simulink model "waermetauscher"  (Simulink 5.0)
settings: Solver=ode45  StartTime=0.0  StopTime=Te  RelTol=1e-3
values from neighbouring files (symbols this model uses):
  A = [0 -1/L; 1/C 0]    [Aufgwok.m]    (also in Behalt.m = [-0.5 0; Bspkran.m = zeros(n, n); Bspmotor.m = [-RA/LA  -km/LA; Bsppend.m = [0  0        1        0)
  c1 = [1 0 0]    [Bsppend.m]    (also in BspSchwinger.m = 0.75; carbrklin.m = 1.2801)
  c2 = 0.4    [BspSchwinger.m]    (also in carbrklin.m = 23.99)
  dt = 0.03    [BodeInterpr.m]    (also in carbrklin.m = 0.01; PerfregSchwinger.m = 0.1; PerfregSchwingkreis.m = 0.0002)
  k = k+1    (= 1)    [Airbag.m]    (also in Bodedia.m = 2; Deltah.m; Fklmotr.m; Laplace.m = 0)
  m1 = 1    [Bsppend.m]    (also in BspSchwinger.m)
  m2 = 1    [BspSchwinger.m]
  w1 = 0.1    [BodeInterpr.m]    (also in FKLLeerlauf.m = 16.7833109017)
  w2 = 1    [BodeInterpr.m]
undefined symbols (not defined in the file or in its folder): deltad, deltaw, T10, T1quer, T20, T2quer

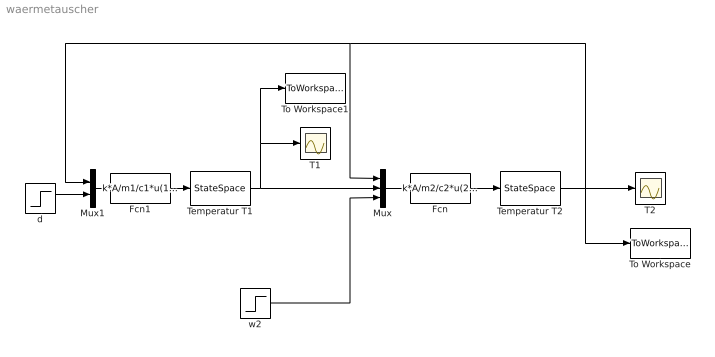
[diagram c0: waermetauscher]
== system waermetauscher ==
  Fcn : Fcn  Expr=k*A/m2/c2*u(2)+T20/m2*u(3)-u(1)*u(3)/m2
  Fcn1 : Fcn  Expr=k*A/m1/c1*u(1)+w1/m1*T10+w1/m1*u(2)
  Mux : Mux  Inputs=3
  Mux1 : Mux  Inputs=2
  T1 : Scope
  T2 : Scope
  Temperatur T1 : StateSpace  A=-w1/m1-k*A/m1/c1  D=0  X0=T1quer
  Temperatur T2 : StateSpace  A=-k*A/m2/c2  D=0  X0=T2quer
  To Workspace : ToWorkspace  VariableName=T2  SampleTime=dt  SaveFormat=Array
  To Workspace1 : ToWorkspace  VariableName=T1  SampleTime=dt  SaveFormat=Array
  d : Step  After=deltad  SampleTime=0
  w2 : Step  Time=2  Before=w2  After=w2+deltaw  SampleTime=0
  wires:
  Mux/1 -> Fcn/1
  w2/1 -> Mux/3
  Fcn/1 -> Temperatur T2/1
  Temperatur T1/1 -> Mux/2, T1/1, To Workspace1/1
  d/1 -> Mux1/2
  Mux1/1 -> Fcn1/1
  Fcn1/1 -> Temperatur T1/1
  Temperatur T2/1 -> T2/1, Mux1/1, Mux/1, To Workspace/1
